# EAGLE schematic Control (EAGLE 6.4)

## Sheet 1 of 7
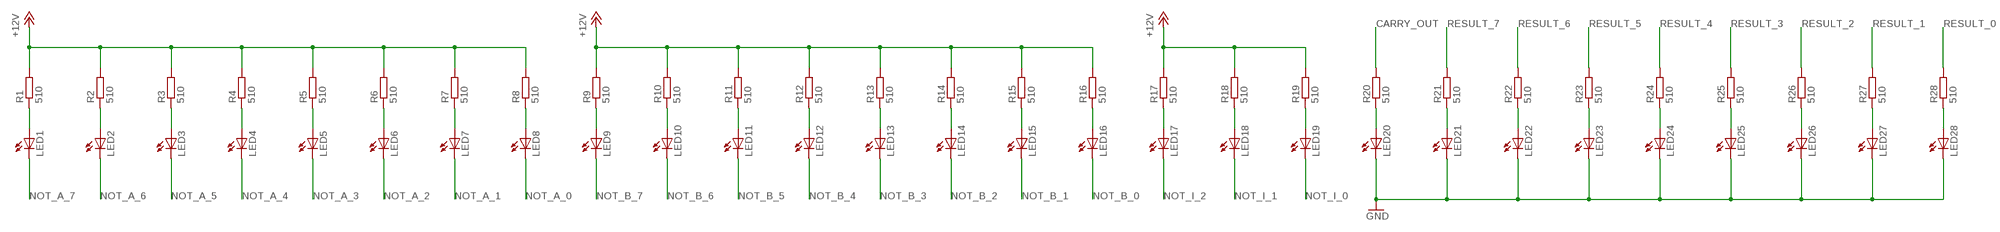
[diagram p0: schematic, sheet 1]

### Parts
LED1  LED5MM  [LED5MM]
LED2  LED5MM  [LED5MM]
LED3  LED5MM  [LED5MM]
LED4  LED5MM  [LED5MM]
LED5  LED5MM  [LED5MM]
LED6  LED5MM  [LED5MM]
LED7  LED5MM  [LED5MM]
LED8  LED5MM  [LED5MM]
LED9  LED5MM  [LED5MM]
LED10  LED5MM  [LED5MM]
LED11  LED5MM  [LED5MM]
LED12  LED5MM  [LED5MM]
LED13  LED5MM  [LED5MM]
LED14  LED5MM  [LED5MM]
LED15  LED5MM  [LED5MM]
LED16  LED5MM  [LED5MM]
LED17  LED5MM  [LED5MM]
LED18  LED5MM  [LED5MM]
LED19  LED5MM  [LED5MM]
LED20  LED5MM  [LED5MM]
LED21  LED5MM  [LED5MM]
LED22  LED5MM  [LED5MM]
LED23  LED5MM  [LED5MM]
LED24  LED5MM  [LED5MM]
LED25  LED5MM  [LED5MM]
LED26  LED5MM  [LED5MM]
LED27  LED5MM  [LED5MM]
LED28  LED5MM  [LED5MM]
R1  510  R  [0207/10]
R2  510  R  [0207/10]
R3  510  R  [0207/10]
R4  510  R  [0207/10]
R5  510  R  [0207/10]
R6  510  R  [0207/10]
R7  510  R  [0207/10]
R8  510  R  [0207/10]
R9  510  R  [0207/10]
R10  510  R  [0207/10]
R11  510  R  [0207/10]
R12  510  R  [0207/10]
R13  510  R  [0207/10]
R14  510  R  [0207/10]
R15  510  R  [0207/10]
R16  510  R  [0207/10]
R17  510  R  [0207/10]
R18  510  R  [0207/10]
R19  510  R  [0207/10]
R20  510  R  [0207/10]
R21  510  R  [0207/10]
R22  510  R  [0207/10]
R23  510  R  [0207/10]
R24  510  R  [0207/10]
R25  510  R  [0207/10]
R26  510  R  [0207/10]
R27  510  R  [0207/10]
R28  510  R  [0207/10]

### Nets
+12V [12V_Power]: R1.2 R2.2 R3.2 R4.2 R5.2 R6.2 R7.2 R8.2 R9.2 R10.2 R11.2 R12.2 R13.2 R14.2 R15.2 R16.2 R17.2 R18.2 R19.2 ; also sheet 5,6,7
CARRY_OUT: R20.2 ; also sheet 2,6
GND [Ground]: LED20.K(C) LED21.K(C) LED22.K(C) LED23.K(C) LED24.K(C) LED25.K(C) LED26.K(C) LED27.K(C) LED28.K(C) ; also sheet 2,3,4,5,6,7
N$2: LED1.A R1.1
N$75: LED2.A R2.1
N$77: LED3.A R3.1
N$78: LED4.A R4.1
N$79: LED5.A R5.1
N$80: LED6.A R6.1
N$81: LED7.A R7.1
N$82: LED8.A R8.1
N$91: LED9.A R9.1
N$92: LED10.A R10.1
N$93: LED11.A R11.1
N$94: LED12.A R12.1
N$95: LED13.A R13.1
N$96: LED14.A R14.1
N$97: LED15.A R15.1
N$98: LED16.A R16.1
N$107: LED17.A R17.1
N$108: LED18.A R18.1
N$109: LED19.A R19.1
N$113: LED20.A R20.1
N$114: LED21.A R21.1
N$115: LED22.A R22.1
N$116: LED23.A R23.1
N$117: LED24.A R24.1
N$118: LED25.A R25.1
N$119: LED26.A R26.1
N$120: LED27.A R27.1
N$129: LED28.A R28.1
NOT_A_0 [Relay_Interconnects]: LED8.K(C) ; also sheet 6,7
NOT_A_1 [Relay_Interconnects]: LED7.K(C) ; also sheet 6,7
NOT_A_2 [Relay_Interconnects]: LED6.K(C) ; also sheet 6,7
NOT_A_3 [Relay_Interconnects]: LED5.K(C) ; also sheet 6,7
NOT_A_4 [Relay_Interconnects]: LED4.K(C) ; also sheet 6,7
NOT_A_5 [Relay_Interconnects]: LED3.K(C) ; also sheet 6,7
NOT_A_6 [Relay_Interconnects]: LED2.K(C) ; also sheet 6,7
NOT_A_7 [Relay_Interconnects]: LED1.K(C) ; also sheet 6,7
NOT_B_0 [Relay_Interconnects]: LED16.K(C) ; also sheet 6,7
NOT_B_1 [Relay_Interconnects]: LED15.K(C) ; also sheet 6,7
NOT_B_2 [Relay_Interconnects]: LED14.K(C) ; also sheet 6,7
NOT_B_3 [Relay_Interconnects]: LED13.K(C) ; also sheet 6,7
NOT_B_4 [Relay_Interconnects]: LED12.K(C) ; also sheet 6,7
NOT_B_5 [Relay_Interconnects]: LED11.K(C) ; also sheet 6,7
NOT_B_6 [Relay_Interconnects]: LED10.K(C) ; also sheet 6,7
NOT_B_7 [Relay_Interconnects]: LED9.K(C) ; also sheet 6,7
NOT_I_0 [Relay_Interconnects]: LED19.K(C) ; also sheet 6,7
NOT_I_1 [Relay_Interconnects]: LED18.K(C) ; also sheet 6,7
NOT_I_2 [Relay_Interconnects]: LED17.K(C) ; also sheet 6,7
RESULT_0: R28.2 ; also sheet 2,6
RESULT_1: R27.2 ; also sheet 2,6
RESULT_2: R26.2 ; also sheet 2,6
RESULT_3: R25.2 ; also sheet 2,6
RESULT_4: R24.2 ; also sheet 2,6
RESULT_5: R23.2 ; also sheet 2,6
RESULT_6: R22.2 ; also sheet 2,6
RESULT_7: R21.2 ; also sheet 2,6

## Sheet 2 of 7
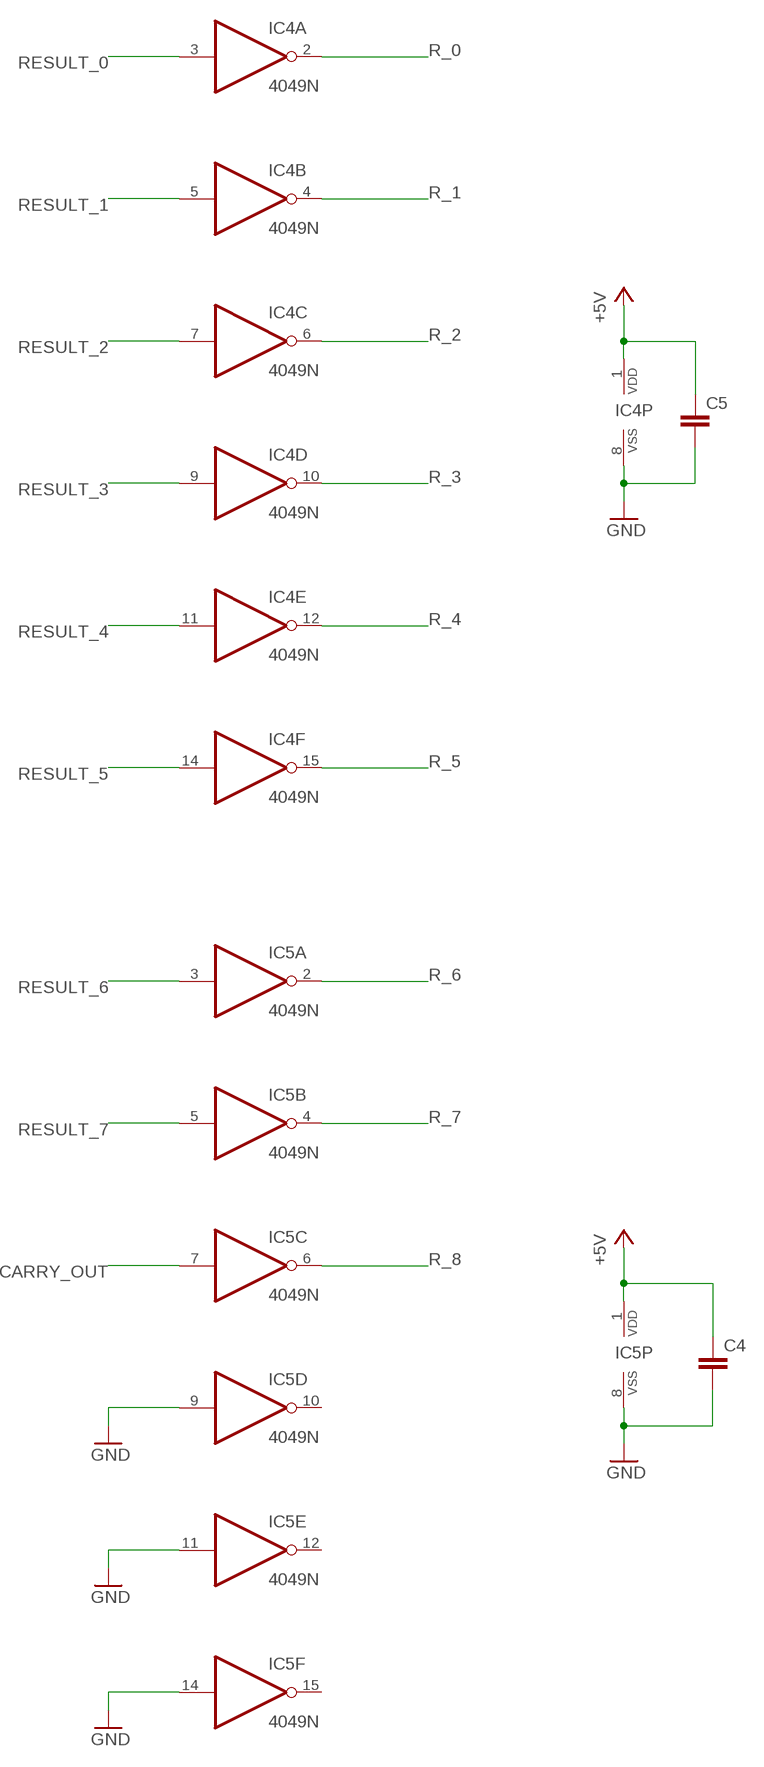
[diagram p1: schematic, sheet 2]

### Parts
C4  C5P  [C050-030-075]
C5  C5P  [C050-030-075]
IC4  4049N  [DIL16]
IC5  4049N  [DIL16]

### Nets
+5V: C4.1 C5.1 IC4.1(P:VDD) IC5.1(P:VDD) ; also sheet 3,4,5
CARRY_OUT: IC5.7(C:I) ; also sheet 1,6
GND [Ground]: C4.2 C5.2 IC4.8(P:VSS) IC5.8(P:VSS) IC5.9(D:I) IC5.11(E:I) IC5.14(F:I) ; also sheet 1,3,4,5,6,7
R_0: IC4.2(A:O) ; also sheet 3
R_1: IC4.4(B:O) ; also sheet 3
R_2: IC4.6(C:O) ; also sheet 3
R_3: IC4.10(D:O) ; also sheet 3
R_4: IC4.12(E:O) ; also sheet 3
R_5: IC4.15(F:O) ; also sheet 3
R_6: IC5.2(A:O) ; also sheet 3
R_7: IC5.4(B:O) ; also sheet 3
R_8: IC5.6(C:O) ; also sheet 3
RESULT_0: IC4.3(A:I) ; also sheet 1,6
RESULT_1: IC4.5(B:I) ; also sheet 1,6
RESULT_2: IC4.7(C:I) ; also sheet 1,6
RESULT_3: IC4.9(D:I) ; also sheet 1,6
RESULT_4: IC4.11(E:I) ; also sheet 1,6
RESULT_5: IC4.14(F:I) ; also sheet 1,6
RESULT_6: IC5.3(A:I) ; also sheet 1,6
RESULT_7: IC5.5(B:I) ; also sheet 1,6
Unconnected: IC5.10(D:O) IC5.12(E:O) IC5.15(F:O)

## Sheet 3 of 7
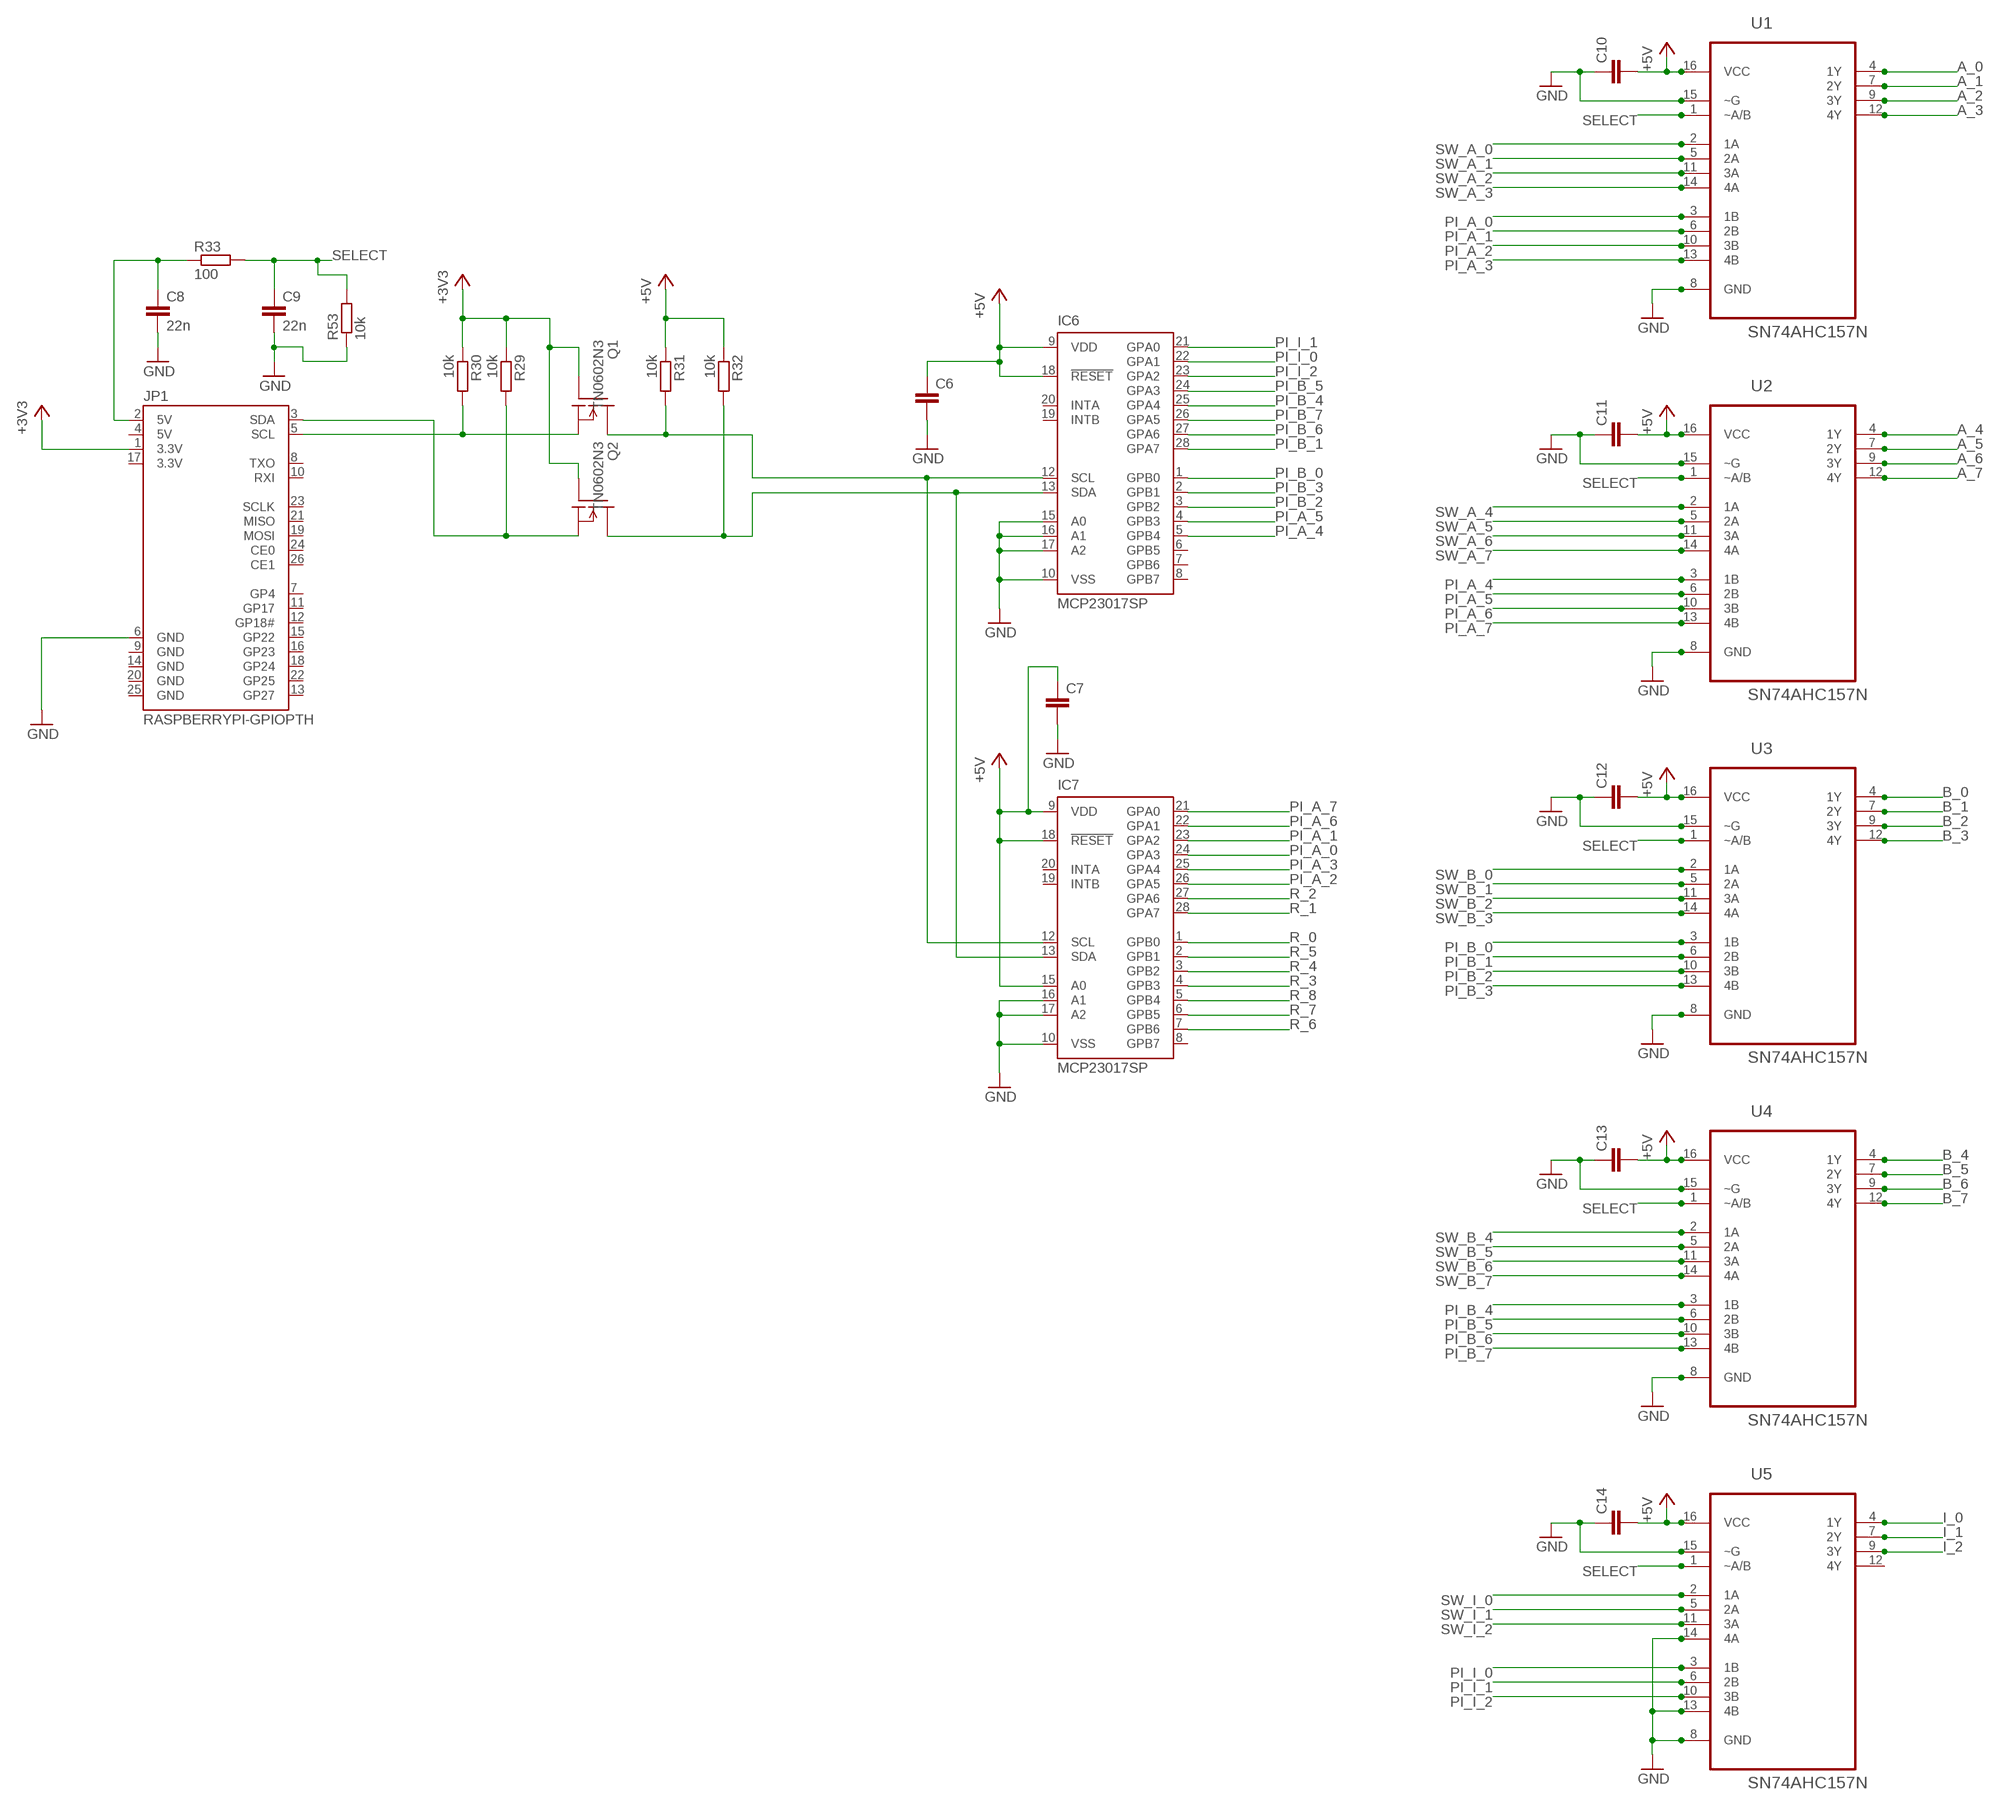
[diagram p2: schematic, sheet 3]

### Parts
C6  C5P  [C050-030-075]
C7  C5P  [C050-030-075]
C8  22n  C5P  [C050-030-075]
C9  22n  C5P  [C050-030-075]
C10  C5P  [C050-030-075]
C11  C5P  [C050-030-075]
C12  C5P  [C050-030-075]
C13  C5P  [C050-030-075]
C14  C5P  [C050-030-075]
IC6  MCP23017SP  [DIL28-3]
IC7  MCP23017SP  [DIL28-3]
JP1  RASPBERRYPI-GPIOPTH  [2X13-SHROUDED]
Q1  TN0602N3  [TO-92]
Q2  TN0602N3  [TO-92]
R29  10k  R  [0207/10]
R30  10k  R  [0207/10]
R31  10k  R  [0207/10]
R32  10k  R  [0207/10]
R33  100  R  [0207/10]
R53  10k  R  [0207/10]
U1  SN74AHC157N  [DIP254P762X508-16]
U2  SN74AHC157N  [DIP254P762X508-16]
U3  SN74AHC157N  [DIP254P762X508-16]
U4  SN74AHC157N  [DIP254P762X508-16]
U5  SN74AHC157N  [DIP254P762X508-16]

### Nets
+3V3: JP1.1(3.3V) Q1.2(G) Q2.2(G) R29.1 R30.1
+5V: C6.1 C7.1 C10.2 C11.2 C12.2 C13.2 C14.2 IC6.9(VDD) IC6.18(!RESET) IC7.9(VDD) IC7.15(A0) IC7.18(!RESET) R31.1 R32.1 U1.16(VCC) U2.16(VCC) U3.16(VCC) U4.16(VCC) U5.16(VCC) ; also sheet 2,4,5
A_0: U1.4(1Y) ; also sheet 7
A_1: U1.7(2Y) ; also sheet 7
A_2: U1.9(3Y) ; also sheet 7
A_3: U1.12(4Y) ; also sheet 7
A_4: U2.4(1Y) ; also sheet 7
A_5: U2.7(2Y) ; also sheet 7
A_6: U2.9(3Y) ; also sheet 7
A_7: U2.12(4Y) ; also sheet 7
B_0: U3.4(1Y) ; also sheet 7
B_1: U3.7(2Y) ; also sheet 7
B_2: U3.9(3Y) ; also sheet 7
B_3: U3.12(4Y) ; also sheet 7
B_4: U4.4(1Y) ; also sheet 7
B_5: U4.7(2Y) ; also sheet 7
B_6: U4.9(3Y) ; also sheet 7
B_7: U4.12(4Y) ; also sheet 7
GND [Ground]: C6.2 C7.2 C8.2 C9.2 C10.1 C11.1 C12.1 C13.1 C14.1 IC6.10(VSS) IC6.15(A0) IC6.16(A1) IC6.17(A2) IC7.10(VSS) IC7.16(A1) IC7.17(A2) JP1.6(GND) R53.1 U1.8(GND) U1.15(~G) U2.8(GND) U2.15(~G) U3.8(GND) U3.15(~G) U4.8(GND) U4.15(~G) U5.8(GND) U5.13(4B) U5.14(4A) U5.15(~G) ; also sheet 1,2,4,5,6,7
I_0: U5.4(1Y) ; also sheet 7
I_1: U5.7(2Y) ; also sheet 7
I_2: U5.9(3Y) ; also sheet 7
N$83: IC6.12(SCL) IC7.12(SCL) Q1.3(D) R31.2
N$84: JP1.5(SCL) Q1.1(S) R30.2
N$85: IC6.13(SDA) IC7.13(SDA) Q2.3(D) R32.2
N$86: JP1.3(SDA) Q2.1(S) R29.2
N$122: C8.1 JP1.2(5V) R33.1
PI_A_0: IC7.24(GPA3) U1.3(1B)
PI_A_1: IC7.23(GPA2) U1.6(2B)
PI_A_2: IC7.26(GPA5) U1.10(3B)
PI_A_3: IC7.25(GPA4) U1.13(4B)
PI_A_4: IC6.5(GPB4) U2.3(1B)
PI_A_5: IC6.4(GPB3) U2.6(2B)
PI_A_6: IC7.22(GPA1) U2.10(3B)
PI_A_7: IC7.21(GPA0) U2.13(4B)
PI_B_0: IC6.1(GPB0) U3.3(1B)
PI_B_1: IC6.28(GPA7) U3.6(2B)
PI_B_2: IC6.3(GPB2) U3.10(3B)
PI_B_3: IC6.2(GPB1) U3.13(4B)
PI_B_4: IC6.25(GPA4) U4.3(1B)
PI_B_5: IC6.24(GPA3) U4.6(2B)
PI_B_6: IC6.27(GPA6) U4.10(3B)
PI_B_7: IC6.26(GPA5) U4.13(4B)
PI_I_0: IC6.22(GPA1) U5.3(1B)
PI_I_1: IC6.21(GPA0) U5.6(2B)
PI_I_2: IC6.23(GPA2) U5.10(3B)
R_0: IC7.1(GPB0) ; also sheet 2
R_1: IC7.28(GPA7) ; also sheet 2
R_2: IC7.27(GPA6) ; also sheet 2
R_3: IC7.4(GPB3) ; also sheet 2
R_4: IC7.3(GPB2) ; also sheet 2
R_5: IC7.2(GPB1) ; also sheet 2
R_6: IC7.7(GPB6) ; also sheet 2
R_7: IC7.6(GPB5) ; also sheet 2
R_8: IC7.5(GPB4) ; also sheet 2
SELECT: C9.1 R33.2 R53.2 U1.1(~A/B) U2.1(~A/B) U3.1(~A/B) U4.1(~A/B) U5.1(~A/B)
SW_A_0: U1.2(1A) ; also sheet 4
SW_A_1: U1.5(2A) ; also sheet 4
SW_A_2: U1.11(3A) ; also sheet 4
SW_A_3: U1.14(4A) ; also sheet 4
SW_A_4: U2.2(1A) ; also sheet 4
SW_A_5: U2.5(2A) ; also sheet 4
SW_A_6: U2.11(3A) ; also sheet 4
SW_A_7: U2.14(4A) ; also sheet 4
SW_B_0: U3.2(1A) ; also sheet 4
SW_B_1: U3.5(2A) ; also sheet 4
SW_B_2: U3.11(3A) ; also sheet 4
SW_B_3: U3.14(4A) ; also sheet 4
SW_B_4: U4.2(1A) ; also sheet 4
SW_B_5: U4.5(2A) ; also sheet 4
SW_B_6: U4.11(3A) ; also sheet 4
SW_B_7: U4.14(4A) ; also sheet 4
SW_I_0: U5.2(1A) ; also sheet 4
SW_I_1: U5.5(2A) ; also sheet 4
SW_I_2: U5.11(3A) ; also sheet 4
Unconnected: IC6.6(GPB5) IC6.7(GPB6) IC6.8(GPB7) IC6.19(INTB) IC6.20(INTA) IC7.8(GPB7) IC7.19(INTB) IC7.20(INTA) JP1.7(GP4) JP1.8(TXO) JP1.10(RXI) JP1.11(GP17) JP1.12(GP18#) JP1.13(GP27) JP1.15(GP22) JP1.16(GP23) JP1.18(GP24) JP1.19(MOSI) JP1.21(MISO) JP1.22(GP25) JP1.23(SCLK) JP1.24(CE0) JP1.26(CE1) U5.12(4Y)

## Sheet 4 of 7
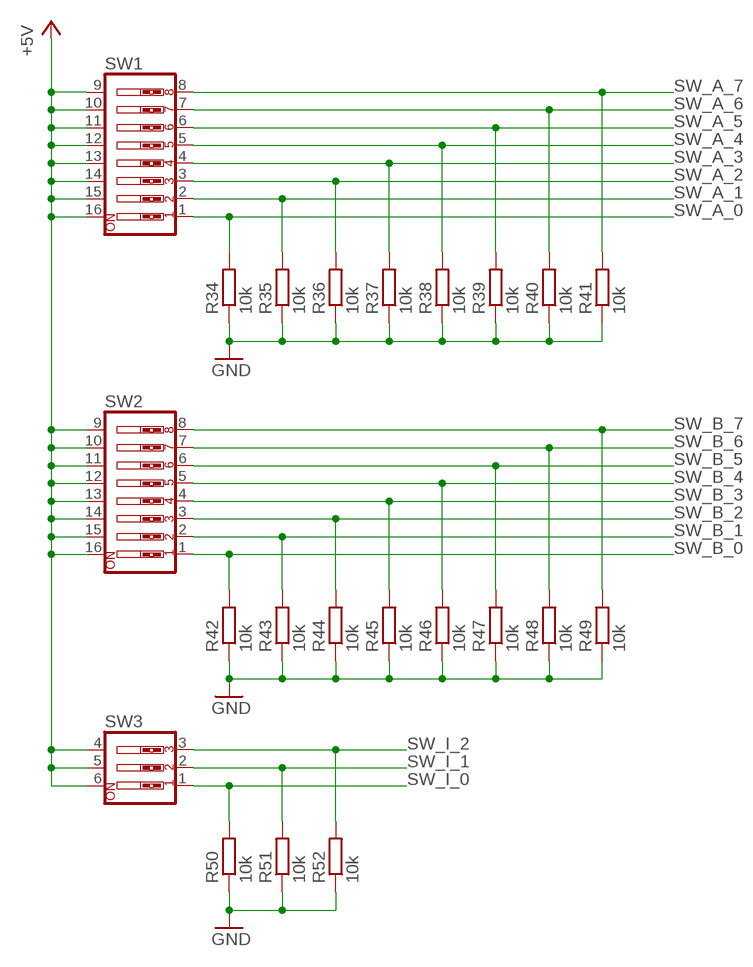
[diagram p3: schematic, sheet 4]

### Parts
R34  10k  R  [0207/10]
R35  10k  R  [0207/10]
R36  10k  R  [0207/10]
R37  10k  R  [0207/10]
R38  10k  R  [0207/10]
R39  10k  R  [0207/10]
R40  10k  R  [0207/10]
R41  10k  R  [0207/10]
R42  10k  R  [0207/10]
R43  10k  R  [0207/10]
R44  10k  R  [0207/10]
R45  10k  R  [0207/10]
R46  10k  R  [0207/10]
R47  10k  R  [0207/10]
R48  10k  R  [0207/10]
R49  10k  R  [0207/10]
R50  10k  R  [0207/10]
R51  10k  R  [0207/10]
R52  10k  R  [0207/10]
SW1  SW_DIP-8  [EDG-08]
SW2  SW_DIP-8  [EDG-08]
SW3  SW_DIP-3  [EDG-03]

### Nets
+5V: SW1.9 SW1.10 SW1.11 SW1.12 SW1.13 SW1.14 SW1.15 SW1.16 SW2.9 SW2.10 SW2.11 SW2.12 SW2.13 SW2.14 SW2.15 SW2.16 SW3.4 SW3.5 SW3.6 ; also sheet 2,3,5
GND [Ground]: R34.1 R35.1 R36.1 R37.1 R38.1 R39.1 R40.1 R41.1 R42.1 R43.1 R44.1 R45.1 R46.1 R47.1 R48.1 R49.1 R50.1 R51.1 R52.1 ; also sheet 1,2,3,5,6,7
SW_A_0: R34.2 SW1.1 ; also sheet 3
SW_A_1: R35.2 SW1.2 ; also sheet 3
SW_A_2: R36.2 SW1.3 ; also sheet 3
SW_A_3: R37.2 SW1.4 ; also sheet 3
SW_A_4: R38.2 SW1.5 ; also sheet 3
SW_A_5: R39.2 SW1.6 ; also sheet 3
SW_A_6: R40.2 SW1.7 ; also sheet 3
SW_A_7: R41.2 SW1.8 ; also sheet 3
SW_B_0: R42.2 SW2.1 ; also sheet 3
SW_B_1: R43.2 SW2.2 ; also sheet 3
SW_B_2: R44.2 SW2.3 ; also sheet 3
SW_B_3: R45.2 SW2.4 ; also sheet 3
SW_B_4: R46.2 SW2.5 ; also sheet 3
SW_B_5: R47.2 SW2.6 ; also sheet 3
SW_B_6: R48.2 SW2.7 ; also sheet 3
SW_B_7: R49.2 SW2.8 ; also sheet 3
SW_I_0: R50.2 SW3.1 ; also sheet 3
SW_I_1: R51.2 SW3.2 ; also sheet 3
SW_I_2: R52.2 SW3.3 ; also sheet 3

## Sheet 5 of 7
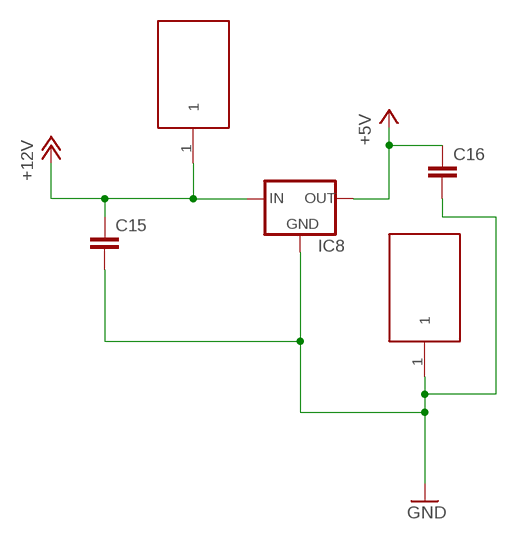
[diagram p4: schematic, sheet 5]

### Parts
C15  C5P  [C050-030-075]
C16  C5P  [C050-030-075]
IC8  78XXS  [78XXS]
U$1  BANANACONNECTOR  [BANPLUG]
U$2  BANANACONNECTOR  [BANPLUG]

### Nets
+5V: C16.1 IC8.OUT ; also sheet 2,3,4
+12V [12V_Power]: C15.1 IC8.IN U$1.1 ; also sheet 1,6,7
GND [Ground]: C15.2 C16.2 IC8.GND U$2.1 ; also sheet 1,2,3,4,6,7

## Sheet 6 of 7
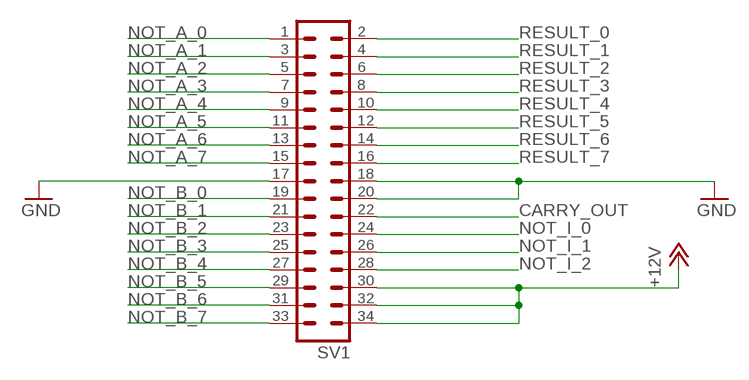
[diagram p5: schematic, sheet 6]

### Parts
SV1  ML34  [ML34]

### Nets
+12V [12V_Power]: SV1.30 SV1.32 SV1.34 ; also sheet 1,5,7
CARRY_OUT: SV1.22 ; also sheet 1,2
GND [Ground]: SV1.17 SV1.18 SV1.20 ; also sheet 1,2,3,4,5,7
NOT_A_0 [Relay_Interconnects]: SV1.1 ; also sheet 1,7
NOT_A_1 [Relay_Interconnects]: SV1.3 ; also sheet 1,7
NOT_A_2 [Relay_Interconnects]: SV1.5 ; also sheet 1,7
NOT_A_3 [Relay_Interconnects]: SV1.7 ; also sheet 1,7
NOT_A_4 [Relay_Interconnects]: SV1.9 ; also sheet 1,7
NOT_A_5 [Relay_Interconnects]: SV1.11 ; also sheet 1,7
NOT_A_6 [Relay_Interconnects]: SV1.13 ; also sheet 1,7
NOT_A_7 [Relay_Interconnects]: SV1.15 ; also sheet 1,7
NOT_B_0 [Relay_Interconnects]: SV1.19 ; also sheet 1,7
NOT_B_1 [Relay_Interconnects]: SV1.21 ; also sheet 1,7
NOT_B_2 [Relay_Interconnects]: SV1.23 ; also sheet 1,7
NOT_B_3 [Relay_Interconnects]: SV1.25 ; also sheet 1,7
NOT_B_4 [Relay_Interconnects]: SV1.27 ; also sheet 1,7
NOT_B_5 [Relay_Interconnects]: SV1.29 ; also sheet 1,7
NOT_B_6 [Relay_Interconnects]: SV1.31 ; also sheet 1,7
NOT_B_7 [Relay_Interconnects]: SV1.33 ; also sheet 1,7
NOT_I_0 [Relay_Interconnects]: SV1.24 ; also sheet 1,7
NOT_I_1 [Relay_Interconnects]: SV1.26 ; also sheet 1,7
NOT_I_2 [Relay_Interconnects]: SV1.28 ; also sheet 1,7
RESULT_0: SV1.2 ; also sheet 1,2
RESULT_1: SV1.4 ; also sheet 1,2
RESULT_2: SV1.6 ; also sheet 1,2
RESULT_3: SV1.8 ; also sheet 1,2
RESULT_4: SV1.10 ; also sheet 1,2
RESULT_5: SV1.12 ; also sheet 1,2
RESULT_6: SV1.14 ; also sheet 1,2
RESULT_7: SV1.16 ; also sheet 1,2

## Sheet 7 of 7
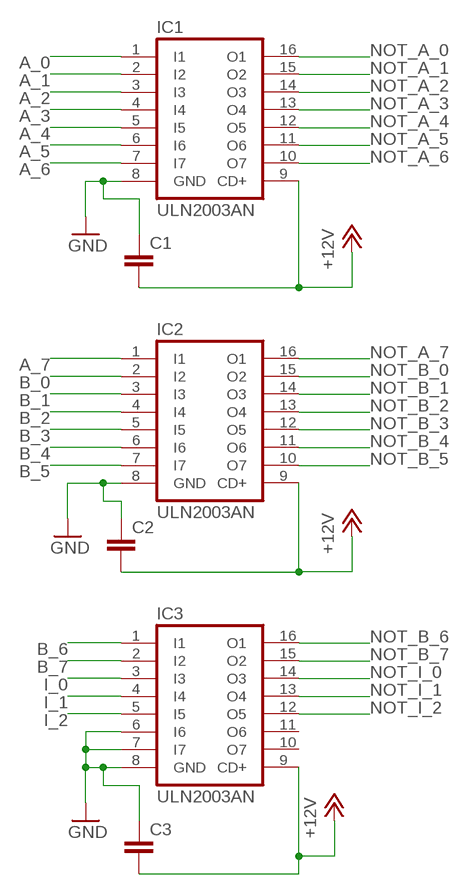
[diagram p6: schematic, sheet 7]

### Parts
C1  C5P  [C050-030-075]
C2  C5P  [C050-030-075]
C3  C5P  [C050-030-075]
IC1  ULN2003AN  [DIL16]
IC2  ULN2003AN  [DIL16]
IC3  ULN2003AN  [DIL16]

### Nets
+12V [12V_Power]: C1.2 C2.2 C3.2 IC1.9(CD+) IC2.9(CD+) IC3.9(CD+) ; also sheet 1,5,6
A_0: IC1.1(I1) ; also sheet 3
A_1: IC1.2(I2) ; also sheet 3
A_2: IC1.3(I3) ; also sheet 3
A_3: IC1.4(I4) ; also sheet 3
A_4: IC1.5(I5) ; also sheet 3
A_5: IC1.6(I6) ; also sheet 3
A_6: IC1.7(I7) ; also sheet 3
A_7: IC2.1(I1) ; also sheet 3
B_0: IC2.2(I2) ; also sheet 3
B_1: IC2.3(I3) ; also sheet 3
B_2: IC2.4(I4) ; also sheet 3
B_3: IC2.5(I5) ; also sheet 3
B_4: IC2.6(I6) ; also sheet 3
B_5: IC2.7(I7) ; also sheet 3
B_6: IC3.1(I1) ; also sheet 3
B_7: IC3.2(I2) ; also sheet 3
GND [Ground]: C1.1 C2.1 C3.1 IC1.8(GND) IC2.8(GND) IC3.6(I6) IC3.7(I7) IC3.8(GND) ; also sheet 1,2,3,4,5,6
I_0: IC3.3(I3) ; also sheet 3
I_1: IC3.4(I4) ; also sheet 3
I_2: IC3.5(I5) ; also sheet 3
NOT_A_0 [Relay_Interconnects]: IC1.16(O1) ; also sheet 1,6
NOT_A_1 [Relay_Interconnects]: IC1.15(O2) ; also sheet 1,6
NOT_A_2 [Relay_Interconnects]: IC1.14(O3) ; also sheet 1,6
NOT_A_3 [Relay_Interconnects]: IC1.13(O4) ; also sheet 1,6
NOT_A_4 [Relay_Interconnects]: IC1.12(O5) ; also sheet 1,6
NOT_A_5 [Relay_Interconnects]: IC1.11(O6) ; also sheet 1,6
NOT_A_6 [Relay_Interconnects]: IC1.10(O7) ; also sheet 1,6
NOT_A_7 [Relay_Interconnects]: IC2.16(O1) ; also sheet 1,6
NOT_B_0 [Relay_Interconnects]: IC2.15(O2) ; also sheet 1,6
NOT_B_1 [Relay_Interconnects]: IC2.14(O3) ; also sheet 1,6
NOT_B_2 [Relay_Interconnects]: IC2.13(O4) ; also sheet 1,6
NOT_B_3 [Relay_Interconnects]: IC2.12(O5) ; also sheet 1,6
NOT_B_4 [Relay_Interconnects]: IC2.11(O6) ; also sheet 1,6
NOT_B_5 [Relay_Interconnects]: IC2.10(O7) ; also sheet 1,6
NOT_B_6 [Relay_Interconnects]: IC3.16(O1) ; also sheet 1,6
NOT_B_7 [Relay_Interconnects]: IC3.15(O2) ; also sheet 1,6
NOT_I_0 [Relay_Interconnects]: IC3.14(O3) ; also sheet 1,6
NOT_I_1 [Relay_Interconnects]: IC3.13(O4) ; also sheet 1,6
NOT_I_2 [Relay_Interconnects]: IC3.12(O5) ; also sheet 1,6
Unconnected: IC3.10(O7) IC3.11(O6)

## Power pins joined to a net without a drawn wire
3.3V: JP1.17(3.3V)
5V: JP1.4(5V)
GND: JP1.9(GND) JP1.14(GND) JP1.20(GND) JP1.25(GND)

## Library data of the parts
C1-C16 = arm-parts:C: Capacitor
IC1-IC3 = uln-udn:ULN2003A: DRIVER ARRAY
IC4 IC5 = 40xx:4049: Hex inverting BUFFER
IC6 IC7 = adafruit:MCP23017: http://ww1.microchip.com/downloads/en/DeviceDoc/21952a.pdf Source: http://ww1.microchip.com/downloads/en/DeviceDoc/21952a.pdf
IC8 = v-reg:78XXS: VOLTAGE REGULATOR
JP1 = SparkFun-Boards:RASPBERRYPI-GPIO: RASPBERRY PI I/O HEADER As defined for the Revistion 2 Pi.; DIST: sparkfun; DIST_ID: PRT-11490
LED1-LED28 = led:LED: LED
Q1 Q2 = transistor-fet:TN0602N3: N-Channel Enhancement MOSFET 20V; 4A; 0,75Ohm
R1-R53 = arm-parts:R: Resistor
SV1 = con-harting-ml:ML34: HARTING; OC_FARNELL: unknown; OC_NEWARK: unknown
SW1 SW2 = special:SW_DIP-8: DIP SWITCH
SW3 = special:SW_DIP-3: DIP SWITCH
U1-U5 = MUX:SN74AHC157N: QUAD 2 LINE TO 1 LINE DATA SELECTORS/MULTIPLEXERS; MPN: SN74AHC157N; OC_FARNELL: 1741531; OC_NEWARK: 34R8444; PACKAGE: 16-DIP; SUPPLIER: Texas Instruments
U$1 U$2 = IR2184:BANANACONNECTOR

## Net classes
1 12V_Power: width 0.762 mm
2 Ground: width 0.762 mm
3 Relay_Interconnects: width 0.762 mm

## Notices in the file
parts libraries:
SparkFun-Boards: Licensing: Creative Commons ShareAlike 4.0 International - https://creativecommons.org/licenses/by-sa/4.0
